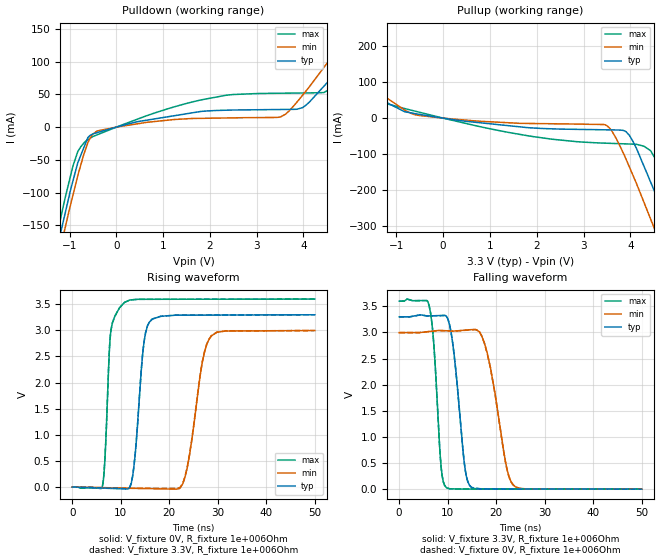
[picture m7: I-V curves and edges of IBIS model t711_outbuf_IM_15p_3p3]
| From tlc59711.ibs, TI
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|   t711_outbuf 3.3V Model with
|   1M ohm and 15 pf load during VT transient
[Model] t711_outbuf_IM_15p_3p3
Model_type   Output
Polarity   Non-Inverting
Vmeas = 1.65
Vref = 1.65
Cref = 15pF
Rref = 1000000
|   typ   min   max
|   (nom PVT)   (Fast PVT)   (slow PVT)
|   ON state : BUFFER OUTPUT TURNED HIGH
C_comp   2.21861E-12   1.89706E-12   2.43266E-12
|   OFF state: BUFFER OUTPUT TURNED LOW
|C_comp   2.16811E-12   2.08969E-12   2.20842E-12
| Where   nom PVT is  Nominal Process, 3.3V, 90C
|   Fast PVT is Strong Process, 3.6V, -40C
|   Slow PVT is Weak Process, 3.0V, 150C
|   C_comp - from L-C Tank method, L = 1nH, peak frequency
| variable   typ   min   max
[Voltage Range]   3.3   3   3.6
|Operating Temperature Range
|   25   85   -40
|Junction Temperature Range
[Temperature Range]   90   150   -40
[Pullup Reference]   3.3   3   3.6
[Pulldown Reference]   0   0   0
[Power Clamp Reference]   3.3   3   3.6
[GND Clamp Reference]   0   0   0
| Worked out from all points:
|   slope of the pulldown table from 0 to 0.495 V, typ, clamps not added: 55.9 ohm
|   slope of the pullup table from 0 to 0.495 V, typ, clamps not added: 55.5 ohm
|   falling waveform, V_fixture 3.3V, R_fixture 1e+006Ohm: 20-80 % time 2ns typ, 3.13ns min, 1.36ns max; typ from 3.3 V to 0 V
|   rising waveform, V_fixture 0V, R_fixture 1e+006Ohm: 20-80 % time 1.62ns typ, 2.68ns min, 1ns max; typ from 0 V to 3.3 V
|   rising waveform, V_fixture 3.3V, R_fixture 1e+006Ohm: 20-80 % time 1.62ns typ, 2.69ns min, 1.02ns max; typ from 0 V to 3.3 V
|   falling waveform, V_fixture 0V, R_fixture 1e+006Ohm: 20-80 % time 2ns typ, 3.13ns min, 1.36ns max; typ from 3.3 V to 0 V
[Pulldown]
|   Voltage   I(typ)   I(min)   I(max)
-3.3V     -930mA     -917.9mA   -959.4mA
-1.237V   -177.4mA   -198.1mA   -154.5mA
-1.096V   -132.4mA   -154.7mA   -108.9mA
-824.5mV  -54.65mA   -74.43mA   -37.49mA
-606.5mV  -15.69mA   -23.59mA   -19.14mA
-421.5mV  -8.589mA   -6.303mA   -12.02mA
1.799V    23.88mA    13.41mA    41.41mA
3.506V    26.93mA    15.5mA     51.78mA
3.978V    29.69mA    48.47mA    52.12mA
4.436V    62.41mA    91.15mA    52.74mA
4.906V    99.09mA    135.9mA    79.97mA
6.59V     238.7mA    296.2mA    190.7mA
[Pullup]
|   Voltage   I(typ)   I(min)   I(max)
-3.3V     211.2mA    252.6mA    158.1mA
-1.761V   85.62mA    106.4mA    59.17mA
-666.6mV  14mA       11.97mA    21.49mA
1.799V    -26.24mA   -14.71mA   -48.61mA
3.435V    -32.26mA   -17.72mA   -69.2mA
3.854V    -34.28mA   -98.24mA   -71.13mA
4.061V    -65.67mA   -159.9mA   -72.07mA
4.521V    -204.2mA   -308.3mA   -109.9mA
4.678V    -258.1mA   -360.9mA   -159.9mA
4.964V    -356.6mA   -459mA     -263.2mA
5.067V    -392mA     -494.4mA   -302.8mA
6.59V     -962.4mA   -1.043A    -910.6mA
[Ramp]
R_load = 1e+006
|   typ   min   max
dV/dt_r   1.97914/1.60885e-009   1.79781/2.67972e-009   2.15968/1.00209e-009
dV/dt_f   1.97917/1.99346e-009   1.79792/3.11365e-009   2.15968/1.35063e-009
[Falling Waveform]
V_fixture = 3.3V
V_fixture_min = 3V
V_fixture_max = 3.6V
R_fixture = 1e+006Ohm
C_fixture = 0F
|   Time   V(typ)   V(min)   V(max)
0s        3.299V     2.997V     3.6V
6.162ns   3.317V     3.018V     3.522V
7.151ns   3.32V      3.029V     2.769V
8.652ns   3.324V     3.037V     429.5mV
9.734ns   3.312V     3.033V     29.88mV
13.59ns   390.8mV    3.044V     3.027mV
14.89ns   35.22mV    3.054V     2.927mV
18.17ns   3.965mV    2.603V     2.674mV
23.45ns   3.382mV    89.53mV    2.266mV
50ns      448.3uV    874.6uV    216.4uV
[Rising Waveform]
V_fixture = 0V
V_fixture_min = 0V
V_fixture_max = 0V
R_fixture = 1e+006Ohm
C_fixture = 0F
|   Time   V(typ)   V(min)   V(max)
0s        269.2uV    595.6uV    87.35uV
6.195ns   -20.41mV   -11.3mV    6.733mV
7.94ns    -26.23mV   -14.65mV   2.975V
10.69ns   -35.42mV   -19.94mV   3.529V
12.42ns   192mV      -23.25mV   3.586V
14.77ns   2.755V     -27.75mV   3.595V
16.46ns   3.212V     -31.01mV   3.595V
22.85ns   3.291V     76.62mV    3.596V
28.68ns   3.293V     2.894V     3.597V
50ns      3.299V     2.997V     3.6V
[Rising Waveform]
V_fixture = 3.3V
V_fixture_min = 3V
V_fixture_max = 3.6V
R_fixture = 1e+006Ohm
C_fixture = 0F
|   Time   V(typ)   V(min)   V(max)
0s        448.3uV    874.6uV    216.4uV
6.191ns   -16.75mV   -11.93mV   7.609mV
7.94ns    -21.62mV   -15.55mV   2.976V
10.69ns   -29.27mV   -21.25mV   3.53V
12.42ns   200.1mV    -24.42mV   3.586V
14.77ns   2.76V      -25.08mV   3.596V
16.46ns   3.213V     -25.56mV   3.596V
22.89ns   3.292V     103.6mV    3.597V
28.66ns   3.293V     2.895V     3.597V
50ns      3.299V     2.997V     3.6V
[Falling Waveform]
|Gnd
V_fixture = 0V
V_fixture_min = 0V
V_fixture_max = 0V
R_fixture = 1e+006Ohm
C_fixture = 0F
|   Time   V(typ)   V(min)   V(max)
0s        3.299V     2.997V     3.6V
6.162ns   3.316V     3.018V     3.521V
7.151ns   3.319V     3.028V     2.768V
8.652ns   3.323V     3.036V     427.9mV
9.734ns   3.31V      3.032V     29.44mV
13.59ns   387.6mV    3.041V     2.792mV
14.89ns   34.39mV    3.05V      2.696mV
18.17ns   3.585mV    2.595V     2.452mV
23.45ns   3.034mV    87.05mV    2.06mV
50ns      269.2uV    595.6uV    87.34uV
